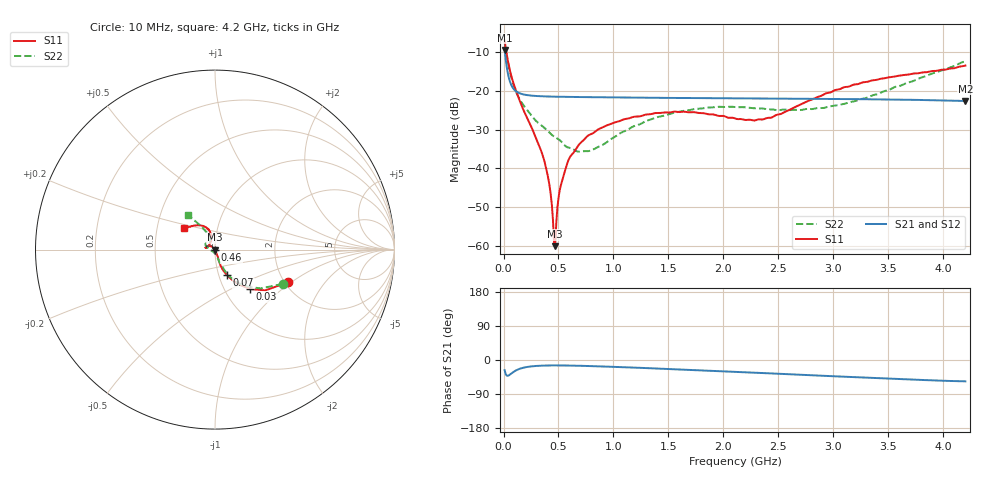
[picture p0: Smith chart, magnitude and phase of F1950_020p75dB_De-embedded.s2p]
! Integrated Device Technology
! Corporate Headquarters
! 6024 Silver Creek Valley Road
! San Jose, CA 95138  USA
! Phone:  1-408-284-8200
! Toll Free:  1-800-223-1366
! Webpage:  http://www.idt.com/
! Timing and RF Division
! 515 Groton Road, Suite 102
! Westford, MA 01886-6024
! Device:  F1950
! Description: 7-bit 0.25 dB Digital Step Attenuator
! Frequency:  150.0 -  4000.00 MHz
! Package:  4x4 mm Thin QFN Plastic Package: 24 pin
! Ports:  2 RF, 12 DC
!  Pin  1  = D0
!  Pin  2  = VDD
!  Pin  3  = Vmode
!  Pin  4  = GND
!  Pin  5  = RF1  =  Port 1
!  Pin  6  = GND
!  Pin  7  = GND
!  Pin  8  = GND
!  Pin  9  = GND
!  Pin 10  = GND
!  Pin 11  = GND
!  Pin 12  = GND
!  Pin 13  = GND
!  Pin 14  = RF2  =  Port 2
!  Pin 15  = GND
!  Pin 16  = LE
!  Pin 17  = CLK
!  Pin 18  = DATE
!  Pin 19  = D6
!  Pin 20  = D5
!  Pin 21  = D4
!  Pin 22  = D3
!  Pin 23  = D2
!  Pin 24  = D1
! State:  83
! Atten State:  20.75 dB
! Voltage:  +5.00 Volts
! Current:  Not Measured mA
! Data:  The device was measured on a the F195X evaluation board which has
!  individual transmission lines to the RF pins.  Data was collected
!  using a calibrated network analyzer.  The evaluation board was
!  de-embedded using a TRL calibration technique.
!  The reference plane is the edge of the package pin.
! Misc:  Board 2019
!  Action Tracker AT0250
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# GHz S dB R 50
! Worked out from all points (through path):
!   420 points, 10 MHz to 4.2 GHz, reference 50 ohm
!   highest |S21| = -9.50 dB at 10 MHz (marker M1); lowest = -22.6 dB at 4.2 GHz (marker M2)
!   group delay of S21, straight-line fit = 28.7 ps
!   lowest |S11| = -60.1 dB at 470 MHz (marker M3), VSWR 1.00, Z = 49.9 + j0.00954 ohm
!   |S11| at or under -10 dB: 26.46 MHz to end of sweep
!   |S22| runs from -35.7 to -7.5 dB; largest |S21 - S12| = 0.00015
!   S11 on the Smith chart (normalised r, x): 10 MHz: 2.08, -0.94; 30 MHz: 1.31, -0.63; 70 MHz: 1.09, -0.32; 460 MHz: 1.00, -0.00; 4.2 GHz: 0.68, +0.17
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0.01  -7.02 -24.1  -9.50 -26.8  -9.50 -26.7  -7.46 -26.8
0.03  -10.63 -48.3  -13.94 -41.2  -13.94 -41.2  -11.27 -48.9
0.07  -16.08 -64.9  -18.49 -35.9  -18.49 -35.9  -16.42 -63.4
0.16  -23.50 -71.1  -20.78 -22.0  -20.78 -22.0  -22.82 -70.5
0.37  -37.95 -65.5  -21.45 -14.7  -21.45 -14.7  -29.52 -77.1
0.42  -44.74 -71.8  -21.49 -14.4  -21.49 -14.4  -30.86 -78.9
0.45  -53.49 -86.3  -21.51 -14.3  -21.51 -14.3  -31.63 -82.6
0.46  -59.29 -112.8  -21.52 -14.3  -21.52 -14.3  -31.84 -84.0
0.47  -60.09 174.5  -21.52 -14.3  -21.52 -14.3  -32.02 -85.5
0.48  -54.09 146.3  -21.53 -14.3  -21.53 -14.3  -32.18 -86.6
0.51  -45.81 136.6  -21.55 -14.3  -21.55 -14.3  -32.72 -88.7
0.56  -40.57 133.1  -21.57 -14.5  -21.57 -14.5  -34.18 -94.5
0.61  -36.84 134.9  -21.59 -14.7  -21.59 -14.7  -34.80 -104.9
0.71  -33.21 136.9  -21.63 -15.4  -21.63 -15.4  -35.64 -124.5
0.99  -28.39 147.2  -21.72 -18.0  -21.72 -18.0  -32.28 -173.4
1.41  -25.75 163.3  -21.82 -22.6  -21.82 -22.6  -26.72 163.9
1.73  -25.51 169.0  -21.87 -26.4  -21.87 -26.4  -24.74 155.2
2.11  -27.19 158.7  -21.95 -31.3  -21.94 -31.4  -24.22 145.4
2.43  -26.95 126.6  -22.00 -35.3  -22.00 -35.3  -24.78 135.1
2.81  -22.20 105.3  -22.07 -40.4  -22.06 -40.4  -24.71 119.7
3.51  -16.51 117.6  -22.24 -49.3  -22.24 -49.4  -19.73 115.5
4.2  -13.50 146.0  -22.65 -56.3  -22.64 -56.4  -12.35 127.9
